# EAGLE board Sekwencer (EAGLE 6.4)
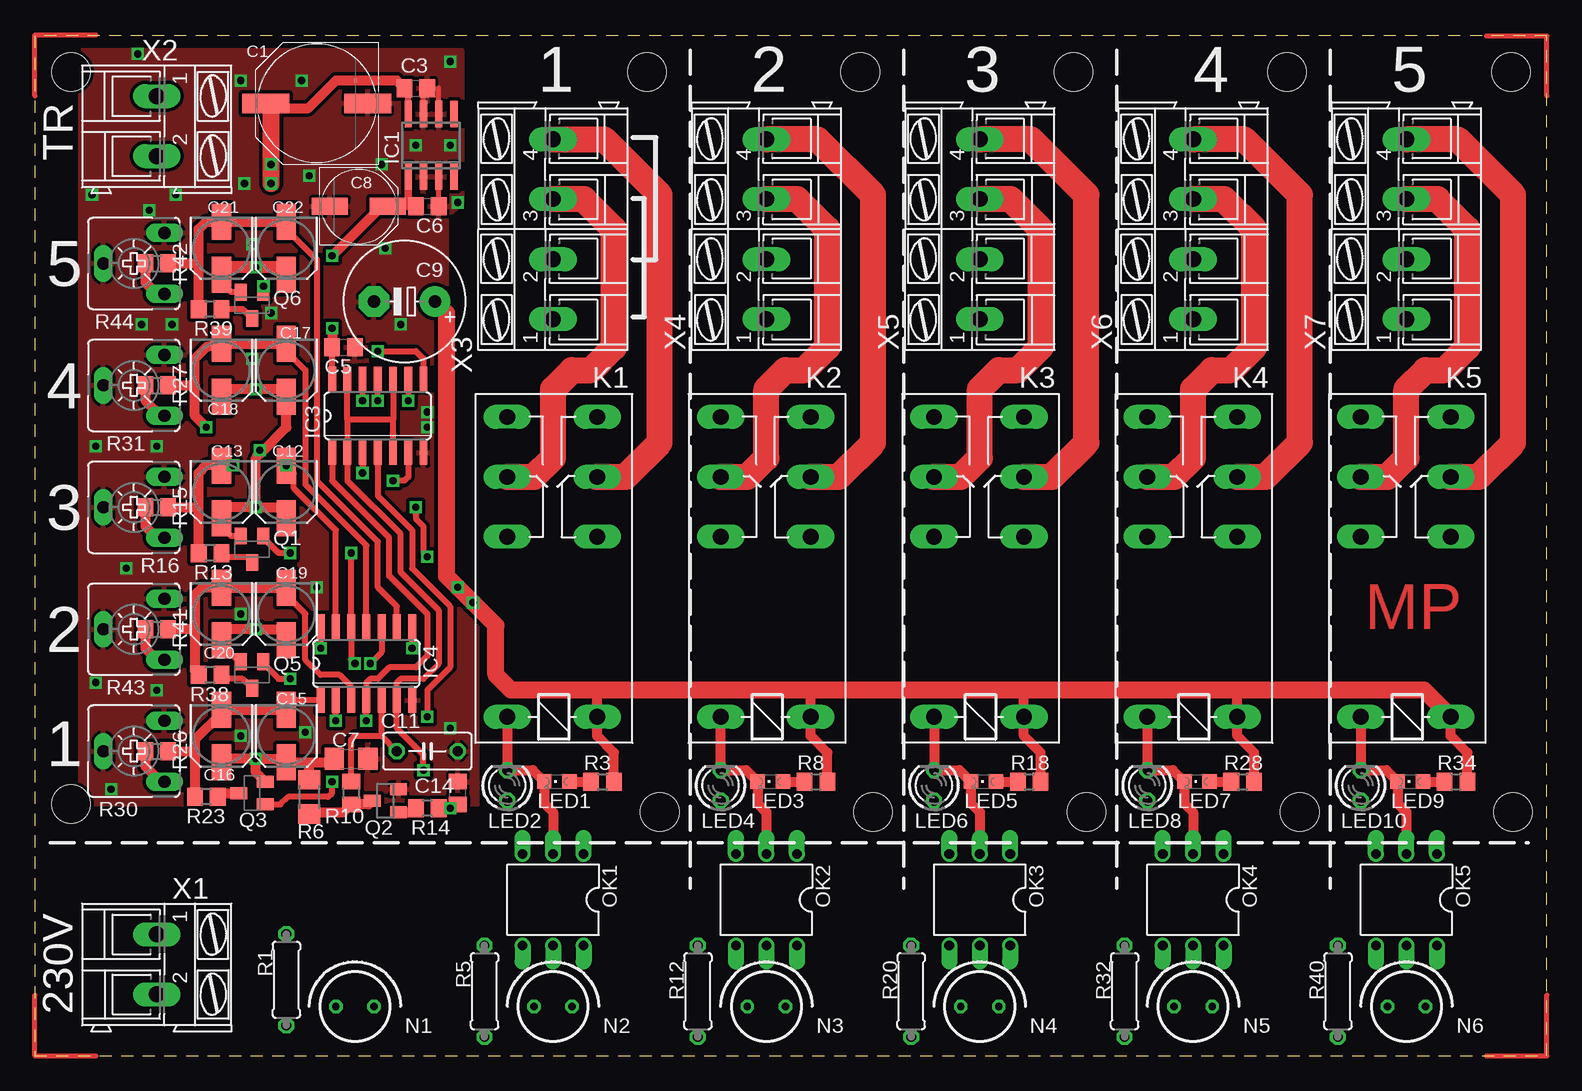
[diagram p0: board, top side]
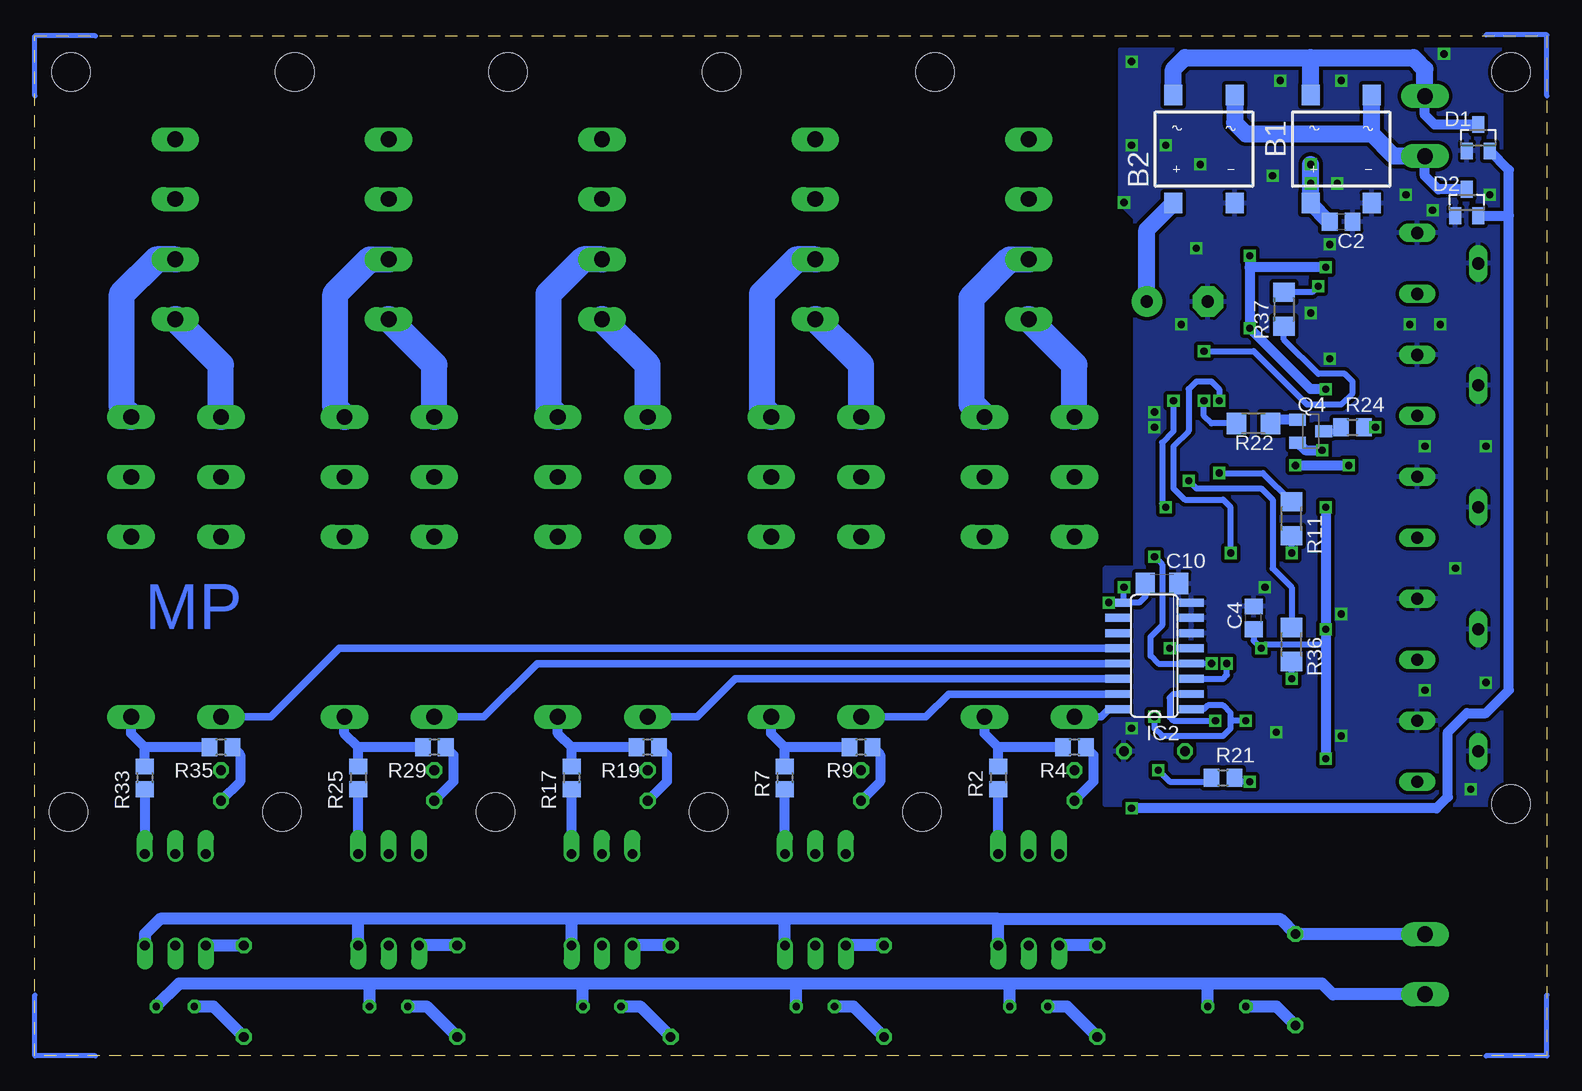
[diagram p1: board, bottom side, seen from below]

Size 126 x 85 mm. Coordinates in mm from the lower left corner, seen from the top.
Outline: 0,0 126,0 126,85 0,85 0,0
Copper layers (1*16): Top 0.035mm / dielectric 1.5mm / Bottom 0.035mm
Design rules "AVT-Elmax": minimum track width 8mil, minimum drill 18mil, track to track 8mil, track to pad 8mil, pad to pad 8mil, via to via 8mil, smd to smd 8mil, copper to edge 10mil, drill to drill 8mil, minimum pad ring 10mil, minimum via ring 8mil, stop-mask expansion 4mil, vias tented up to drill 0mil, thermal gap 10mil
Holes 3.2 mm at 52.07,20.32 69.85,20.32 87.63,20.32 105.41,20.32 123.19,20.32 51,82 68.78,82 86.56,82 104.34,82 123,82 3,82 3,21

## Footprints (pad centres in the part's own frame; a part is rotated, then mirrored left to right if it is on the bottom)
DFS = smd 1.5 x 1.7: + -2.55,-4.5; - 2.55,-4.5; AC1 -2.55,4.5; AC2 2.55,4.5
PANASONIC_G = smd 3.9 x 1.6: + 4.25,0; - -4.25,0
C0805 = smd 1.3 x 1.5: 1 -0.95,0; 2 0.95,0
C1206 = smd 1.6 x 1.8: 1 -1.4,0; 2 1.4,0
PANASONIC_D = smd 3 x 1.4: + 2.4,0; - -2.4,0
E5-10,5 = drill 1.016 pad 2.54: + -2.54,0 | drill 1.016 pad 2.54 octagon: - 2.54,0
C050-030X075 = drill 0.813 octagon: 1 -2.54,0; 2 2.54,0
SANYO-OSCON_SMD_B6 = smd 3 x 1.6: + 2.2,0; - -2.2,0
SOT23 = smd 1 x 1.4: 1 -0.95,-1.1; 2 0.95,-1.1; 3 0,1.1
SO-08 = smd 0.6 x 2.2: 1 -1.905,-2.6; 2 -0.635,-2.6; 3 0.635,-2.6; 4 1.905,-2.6; 5 1.905,2.6; 6 0.635,2.6; 7 -0.635,2.6; 8 -1.905,2.6
SO16 = smd 0.66 x 2.032: 1 -4.445,-3.073; 2 -3.175,-3.073; 3 -1.905,-3.073; 4 -0.635,-3.073; 5 0.635,-3.073; 6 1.905,-3.073; 7 3.175,-3.073; 8 4.445,-3.073; 9 4.445,3.073; 10 3.175,3.073; 11 1.905,3.073; 12 0.635,3.073; 13 -0.635,3.073; 14 -1.905,3.073; 15 -3.175,3.073; 16 -4.445,3.073
SO14 = smd 0.66 x 2.032: 1 -3.81,-3.073; 2 -2.54,-3.073; 3 -1.27,-3.073; 4 0,-3.073; 5 1.27,-3.073; 6 2.54,-3.073; 7 3.81,-3.073; 8 3.81,3.073; 9 2.54,3.073; 10 1.27,3.073; 11 0,3.073; 12 -1.27,3.073; 13 -2.54,3.073; 14 -3.81,3.073
G2R2 = drill 1.321 long: 1 -2.54,-3.683; 2 -2.54,3.81; O1 12.471,3.81; O2 12.471,-3.683; P1 17.45,3.81; P2 17.45,-3.683; S1 22.454,3.81; S2 22.454,-3.683
CHIPLED_0805 = smd 1.2 x 1.2: A 0,-1.05; C 0,1.05
LED3MM = drill 0.813 octagon: A -1.27,0; K 1.27,0
IN-3 = drill 0.6 octagon: A -1.587,0; K 1.587,0
DIL06 = drill 0.813 offset: 1 -2.54,-3.81; 2 0,-3.81; 3 2.54,-3.81; 4 2.54,3.81; 5 0,3.81; 6 -2.54,3.81
SOT23-BEC = smd 1 x 1.4: B -0.95,-1.1; C 0,1.1; E 0.95,-1.1
0207/7 = drill 0.813 octagon: 1 -3.81,0; 2 3.81,0
R0805 = smd 1.3 x 1.5: 1 -0.95,0; 2 0.95,0
R1206 = smd 1.6 x 1.803: 1 -1.422,0; 2 1.422,0
CA6V = drill 1.016 long: A -2.54,-2.54; E 2.54,-2.54; S 0,2.54
AK300/2 = drill 1.321 long: 1 -2.515,0; 2 2.489,0
AK300/4 = drill 1.321 long: 1 -7.493,0; 2 -2.515,0; 3 2.515,0; 4 7.493,0

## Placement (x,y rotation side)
B1  DF06S  [DFS]  17.14,75.56 0 bottom
B2  DF06S  [DFS]  28.57,75.56 0 bottom
C1  470u  [PANASONIC_G]  23.5,79.38 180 top
C2  100n  [C0805]  17.14,69.53 0 bottom
C3  100n  [C0805]  31.75,80.64 0 top
C4  100n  [C0805]  24.45,36.51 90 bottom
C5  100n  [C0805]  25.72,59.05 0 top
C6  100n  [C0805]  32.7,70.8 0 top
C7  100n  [C1206]  26.35,24.77 0 top
C8  100u  [PANASONIC_D]  26.99,70.8 0 top
C9  1000u  [E5-10,5]  30.8,62.87 180 top
C10  100n  [C1206]  32.07,39.37 0 bottom
C11  100n  [C050-030X075]  32.7,25.4 0 top
C12  22u  [SANYO-OSCON_SMD_B6]  20.95,46.99 270 top
C13  22u  [SANYO-OSCON_SMD_B6]  15.56,46.99 270 top
C14  100n  [C0805]  35.24,21.91 90 top
C15  22u  [SANYO-OSCON_SMD_B6]  20.95,26.67 270 top
C16  22u  [SANYO-OSCON_SMD_B6]  15.56,26.67 270 top
C17  22u  [SANYO-OSCON_SMD_B6]  20.95,57.15 270 top
C18  22u  [SANYO-OSCON_SMD_B6]  15.56,57.15 270 top
C19  22u  [SANYO-OSCON_SMD_B6]  20.95,36.83 270 top
C20  22u  [SANYO-OSCON_SMD_B6]  15.56,36.83 270 top
C21  22u  [SANYO-OSCON_SMD_B6]  15.56,67.31 270 top
C22  22u  [SANYO-OSCON_SMD_B6]  20.95,67.31 270 top
D1  BAV99  [SOT23]  5.71,76.52 0 bottom
D2  BAV99  [SOT23]  6.67,71.12 0 bottom
IC1  LM2931-5  [SO-08]  33.02,75.88 0 top
IC2  ULN2003  [SO16]  32.7,33.34 90 bottom
IC3  74HC08  [SO14]  28.57,53.34 0 top
IC4  74HC14  [SO14]  27.62,32.7 0 top
K1  RM83  [G2R2]  43.18,30.8 90 top
K2  RM83  [G2R2]  60.96,30.8 90 top
K3  RM83  [G2R2]  78.74,30.8 90 top
K4  RM83  [G2R2]  96.52,30.8 90 top
K5  RM83  [G2R2]  114.3,30.8 90 top
LED1  [CHIPLED_0805]  43.5,22.86 90 top
LED2  [LED3MM]  39.37,22.54 90 top
LED3  [CHIPLED_0805]  61.28,22.86 90 top
LED4  [LED3MM]  57.15,22.54 90 top
LED5  [CHIPLED_0805]  79.06,22.86 90 top
LED6  [LED3MM]  74.93,22.54 90 top
LED7  [CHIPLED_0805]  96.84,22.86 90 top
LED8  [LED3MM]  92.71,22.54 90 top
LED9  [CHIPLED_0805]  114.62,22.86 90 top
LED10  [LED3MM]  110.49,22.54 90 top
N1  IN-3  [IN-3]  26.67,4.13 0 top
N2  IN-3  [IN-3]  43.18,4.13 0 top
N3  IN-3  [IN-3]  60.96,4.13 0 top
N4  IN-3  [IN-3]  78.74,4.13 0 top
N5  IN-3  [IN-3]  96.52,4.13 0 top
N6  IN-3  [IN-3]  114.3,4.13 0 top
OK1  MOC3041M  [DIL06]  43.18,13.02 180 top
OK2  MOC3041M  [DIL06]  60.96,13.02 180 top
OK3  MOC3041M  [DIL06]  78.74,13.02 180 top
OK4  MOC3041M  [DIL06]  96.52,13.02 180 top
OK5  MOC3041M  [DIL06]  114.3,13.02 180 top
Q1  BC807-40  [SOT23-BEC]  18.1,42.23 180 top
Q2  BC846  [SOT23]  29.21,21.27 90 top
Q3  BC807-40  [SOT23-BEC]  18.1,21.91 90 top
Q4  BC807-40  [SOT23-BEC]  19.68,52.07 270 bottom
Q5  BC807-40  [SOT23-BEC]  18.1,31.75 180 top
Q6  BC807-40  [SOT23-BEC]  18.1,62.55 180 top
R1  220k  [0207/7]  20.95,6.35 270 top
R2  1k  [R0805]  45.72,23.18 270 bottom
R3  2k2  [R0805]  47.31,22.86 0 top
R4  *  [R0805]  39.37,25.72 180 bottom
R5  220k  [0207/7]  37.47,5.4 270 top
R6  51k  [R1206]  22.86,21.59 90 top
R7  1k  [R0805]  63.5,23.18 270 bottom
R8  2k2  [R0805]  65.09,22.86 0 top
R9  *  [R0805]  57.15,25.72 180 bottom
R10  100  [R0805]  26.35,21.91 270 top
R11  2k2  [R1206]  21.27,44.77 270 bottom
R12  220k  [0207/7]  55.24,5.4 270 top
R13  100  [R0805]  14.61,41.91 180 top
R14  10k  [R0805]  32.7,20.64 180 top
R15  10k  [R0805]  10.16,45.72 0 top
R16  1M  [CA6V]  8.26,45.72 90 top
R17  1k  [R0805]  81.28,23.18 270 bottom
R18  2k2  [R0805]  82.87,22.86 0 top
R19  *  [R0805]  74.93,25.72 180 bottom
R20  220k  [0207/7]  73.03,5.4 270 top
R21  2k2  [R0805]  26.99,23.18 0 bottom
R22  2k2  [R1206]  24.45,52.7 0 bottom
R23  100  [R0805]  14.29,21.59 180 top
R24  100  [R0805]  16.19,52.39 0 bottom
R25  1k  [R0805]  99.06,23.18 270 bottom
R26  10k  [R0805]  10.16,25.4 0 top
R27  10k  [R0805]  10.16,55.88 0 top
R28  2k2  [R0805]  100.65,22.86 0 top
R29  *  [R0805]  92.71,25.72 180 bottom
R30  1M  [CA6V]  8.26,25.4 90 top
R31  1M  [CA6V]  8.26,55.88 90 top
R32  220k  [0207/7]  90.81,5.4 270 top
R33  1k  [R0805]  116.84,23.18 270 bottom
R34  2k2  [R0805]  118.43,22.86 0 top
R35  *  [R0805]  110.49,25.72 180 bottom
R36  2k2  [R1206]  21.27,34.29 270 bottom
R37  2k2  [R1206]  21.91,62.23 90 bottom
R38  100  [R0805]  14.61,31.75 180 top
R39  100  [R0805]  14.61,62.23 180 top
R40  220k  [0207/7]  108.58,5.4 270 top
R41  10k  [R0805]  10.16,35.56 0 top
R42  10k  [R0805]  10.16,66.04 0 top
R43  1M  [CA6V]  8.26,35.56 90 top
R44  1M  [CA6V]  8.26,66.04 90 top
X1  230V  [AK300/2]  10.16,7.62 270 top
X2  TR  [AK300/2]  10.16,77.47 270 top
X3  [AK300/4]  43.18,68.9 90 top
X4  [AK300/4]  60.96,68.9 90 top
X5  [AK300/4]  78.74,68.9 90 top
X6  [AK300/4]  96.52,68.9 90 top
X7  [AK300/4]  114.3,68.9 90 top

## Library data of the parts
B1 B2 = rectifier
C1-C22 R1-R15 R17-R29 R32-R42 = rcl
D1 D2 = diode
IC1 = v-reg
IC2 = uln-udn
IC3 IC4 = 74xx-eu
K1-K5 = relay; MF: OMRON COMPONENTS USA; MPN: G2R-2-DC6; OC_FARNELL: unknown; OC_NEWARK: 89C5317
LED1-LED10 = led
N1-N6 = russian-nixies
OK1-OK5 = optocoupler; MF: FAIRCHILD SEMICONDUCTOR; MPN: MOC3041M; OC_FARNELL: 1086677; OC_NEWARK: 78K6090
Q1 Q3-Q6 = transistor-pnp
Q2 = transistor-npn
R16 R30 R31 R43 R44 = pot
X1-X7 = con-ptr500; OC_FARNELL: unknown; OC_NEWARK: unknown

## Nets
!RESET: IC3.2 IC3.5 IC3.10 IC3.13 IC4.6 R21.1
+5V: C4.1 C5.1 C6.1 C7.1 C8.+ C12.+ C13.+ C15.+ C16.+ C17.+ C18.+ C19.+ C20.+ C21.+ C22.+ IC1.1 IC3.14 IC4.14 Q1.E Q3.E Q4.E Q5.E Q6.E R6.2
GND: B1.- B2.- C1.- C2.2 C3.2 C4.2 C5.2 C6.2 C7.2 C8.- C9.- C10.2 C11.2 C14.2 D1.1 D2.1 IC1.2 IC1.3 IC1.6 IC1.7 IC2.6 IC2.7 IC2.8 IC3.7 IC4.7 Q2.2 R16.E R16.S R30.E R30.S R31.E R31.S R43.E R43.S R44.E R44.S
N$1: B1.AC1 B2.AC1 D1.3 X2.1
N$2: B1.AC2 B2.AC2 D2.3 X2.2
N$3: OK1.1 R2.2
N$4: K1.S1 X3.1
N$5: B1.+ C1.+ C2.1 C3.1 IC1.8
N$6: N1.A R1.2
N$7: LED1.A R3.1
N$8: LED2.A R4.1
N$9: Q2.1 R14.2
N$10: C14.1 D1.2 D2.2 R14.1
N$11: Q2.3 R6.1 R10.2
N$12: C15.- C16.- IC4.1 R23.2 R26.2
N$13: Q3.B R21.2
N$14: C19.- C20.- IC4.3 R38.2 R41.2
N$15: IC3.6 R36.1
N$16: Q5.B R36.2
N$17: R41.1 R43.A
N$18: IC3.3 R11.1
N$19: Q1.B R11.2
N$20: C12.- C13.- IC4.13 R13.2 R15.2
N$21: R15.1 R16.A
N$22: IC3.11 R22.1
N$23: Q4.B R22.2
N$24: C17.- C18.- IC4.11 R24.2 R27.2
N$25: R27.1 R31.A
N$26: Q6.B R37.2
N$27: C21.- C22.- IC4.9 R39.2 R42.2
N$28: R42.1 R44.A
N$29: IC3.8 R37.1
N$30: R26.1 R30.A
N$31: K1.P1 X3.3
N$32: K1.P2 X3.4
N$33: K1.S2 X3.2
N$34: OK1.4 R5.1
N$35: N2.A R5.2
N$36: K2.P2 X4.4
N$37: K2.S1 X4.1
N$38: K2.S2 X4.2
N$39: K2.P1 X4.3
N$40: OK2.4 R12.1
N$41: N3.A R12.2
N$42: LED4.A R9.1
N$43: LED3.A R8.1
N$45: OK2.1 R7.2
N$46: OK3.1 R17.2
N$47: K3.S1 X5.1
N$48: LED6.A R19.1
N$49: LED5.A R18.1
N$50: K4.P2 X6.4
N$52: OK3.4 R20.1
N$53: N4.A R20.2
N$54: K3.P2 X5.4
N$55: K3.S2 X5.2
N$56: K3.P1 X5.3
N$57: K4.S1 X6.1
N$58: K4.S2 X6.2
N$59: K4.P1 X6.3
N$60: OK4.4 R32.1
N$61: N5.A R32.2
N$62: LED8.A R29.1
N$63: LED7.A R28.1
N$65: OK4.1 R25.2
N$66: OK5.1 R33.2
N$67: LED10.A R35.1
N$68: LED9.A R34.1
N$70: OK5.4 R40.1
N$71: N6.A R40.2
N$72: K5.P2 X7.4
N$73: K5.S2 X7.2
N$74: K5.P1 X7.3
N$75: K5.S1 X7.1
N$76: N1.K N2.K N3.K N4.K N5.K N6.K X1.2
N$77: OK1.6 OK2.6 OK3.6 OK4.6 OK5.6 R1.1 X1.1
N$82: Q6.C R39.1
N$83: Q4.C R24.1
N$84: Q1.C R13.1
N$85: Q5.C R38.1
N$86: Q3.C R23.1
N$87: C11.1 IC4.5 R10.1
OC1: IC2.16 K1.2 LED1.C LED2.K OK1.2
OC2: IC2.15 K2.2 LED3.C LED4.K OK2.2
OC3: IC2.14 K3.2 LED5.C LED6.K OK3.2
OC4: IC2.13 K4.2 LED7.C LED8.K OK4.2
OC5: IC2.12 K5.2 LED9.C LED10.K OK5.2
REL1: IC2.1 IC3.4 IC4.2
REL2: IC2.2 IC3.1 IC4.4
REL3: IC2.3 IC3.12 IC4.12
REL4: IC2.4 IC3.9 IC4.10
REL5: IC2.5 IC4.8
VCC: B2.+ C9.+ C10.1 IC2.9 K1.1 K2.1 K3.1 K4.1 K5.1 R2.1 R3.2 R4.2 R7.1 R8.2 R9.2 R17.1 R18.2 R19.2 R25.1 R28.2 R29.2 R33.1 R34.2 R35.2

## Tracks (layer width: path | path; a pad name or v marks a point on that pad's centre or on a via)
!RESET  (via drill 0.6)
  Top 0.508: 26.04,53.02 IC3.13 | IC3.10 29.84,53.02 | 29.84,53.02 26.04,53.02 | IC3.5 29.84,53.02 | 26.04,53.02 IC3.2 26.04,47.94 30.48,43.5 30.48,40.32 33.66,37.15 33.66,32.7 32.38,31.43 30.48,31.43 30.16,31.11 IC4.6 30.16,27.3 32.38,25.08 v32.38,23.81
  Bottom 0.508: v32.38,23.81 31.43,22.86 28.25,22.86 R21.1
+5V  (via drill 0.6, 0.6 pad 0.25)
  Top 0.508: IC4.14 v23.81,33.97 | IC3.14 C5.1 | Q1.E 16.36,43.33 15.56,44.13 C13.+ | Q5.E 17,32.85 15.56,34.29 C20.+ | Q6.E 16.36,63.65 15.56,64.45 C21.+
  Top 0.61: C8.+ 31.11,70.8 | 31.11,70.8 C6.1 | IC1.1 31.11,70.8
  Top 0.813: v24.77,60.64 C5.1 | 18.41,45.71 v18.41,45.72 18.41,49.85 18.89,50.32 | v18.41,55.55 v18.41,55.56 | v24.77,66.67 28.89,70.8 C8.+ | v18.41,55.56 15.85,55.56 C18.+ | v18.41,55.56 20.66,55.56 C17.+ 20.95,52.39 18.89,50.32 | 18.41,45.71 15.56,45.71 C13.+ | 18.41,45.71 20.95,45.71 C12.+ | v18.73,50.48 18.89,50.32 | C20.+ 15.56,35.55 v18.41,35.55 20.95,35.55 C19.+ | v18.41,24.77 15.85,24.77 C16.+ | v18.41,24.77 20.02,24.77 C15.+ 22.86,24.47 | 22.86,24.47 24.66,24.47 C7.1 | R6.2 22.86,24.47 | Q3.E 18.41,23.64 v18.41,24.77
  Top 1.016: C22.+ 20.93,65.72 v18.41,65.72 15.58,65.72 C21.+
  Bottom 0.508: 18.41,33.97 18.41,34.29 23.5,34.29 v23.81,33.97 24.45,34.61 C4.1 | Q4.E
  Bottom 0.813: v24.77,66.67 24.77,65.72 | 24.77,65.72 v24.77,60.64 19.68,55.56 v18.41,55.56 | v18.41,45.72 v18.41,35.55 18.41,33.97 v18.41,24.77 | v18.41,65.72 24.77,65.72 | Q4.E 20.15,50.48 v18.73,50.48
GND  (via drill 0.6)
  Top 0.406: 33.66,78.42 33.66,80.64 | 32.38,78.74 32.38,80.64 | 33.66,71.12 33.66,73.03
  other vias: 32.7,53.66 32.7,52.39 5.08,31.11 10.16,30.48 7.62,40.64 5.08,50.8 10.16,50.8 8.89,60.96 11.43,60.96 9.53,70.48 29.21,67.31 30.48,60.96 28.89,74.3 34.61,82.87 22.23,81.28 22.54,26.99 11.75,71.75 34.61,75.88 31.75,75.88 34.61,27.3 17.46,72.71 17.14,81.28 22.86,73.34 18.1,67.63 8.57,83.5 35.24,71.12 4.76,71.75 6.35,22.23 19.68,61.91 18.1,58.1 23.5,39.05 17.14,36.83 17.14,26.67
  pour Top (isolate 0.305): 3.81,83.82 35.56,83.82 35.56,71.12 34.29,69.85 34.29,40.64 36.83,40.64 36.83,20.95 3.81,20.95
  pour Bottom (isolate 0.305): 3.81,83.82 35.56,83.82 35.56,71.12 34.29,69.85 34.29,40.64 36.83,40.64 36.83,20.95 3.81,20.95
N$1
  Bottom 0.813: 9.99,82.06 10.16,82.23 | D1.3 9.36,77.62 10.16,78.42 X2.1
  Bottom 1.422: X2.1 10.16,82.23 11.11,83.19 19.68,83.19 | B2.AC1 31.12,82.22 30.16,83.19 19.68,83.19 | B1.AC1 19.7,82.54 19.68,83.19
N$2
  Bottom 0.813: D2.3 9.04,72.22 10.16,73.34 X2.2
  Bottom 1.422: X2.2 12.75,74.98 14.61,76.83 | 14.61,76.83 14.61,80.06 B1.AC2 | B2.AC2 26.02,77.78 25.08,76.83 14.61,76.83
N$3
  Bottom 0.813: OK1.1 R2.2
N$4
  Bottom 2.184: K1.S1 39.37,57.59 X3.1
N$5  (via drill 0.6)
  Top 0.508: IC1.8 31.11,80.33 C3.1
  Top 0.813: C3.1 30.16,81.28 25.08,81.28 22.74,78.94 19.68,78.94
  Top 1.422: v19.68,72.71 v19.68,74.3 19.68,78.94 C1.+
  Bottom 1.27: C2.1 18.16,69.53 B1.+
  Bottom 1.422: B1.+ 19.7,72.08 v19.68,72.71 v19.68,74.3
N$6
  Bottom 1.016: N1.A 22.54,4.13 R1.2
N$7
  Top 0.813: LED1.A R3.1
N$8
  Bottom 0.813: R4.1 37.78,25.08 37.78,22.86 LED2.A
N$9
  Top 0.813: Q2.1 31.44,20.32 R14.2
N$10  (via drill 0.6)
  Top 0.508: R14.1 33.65,20.32
  Top 0.813: 33.65,20.32 33.66,20.32 | R14.1 v34.61,20.64 34.93,20.96 C14.1
  Bottom 0.813: v34.61,20.64 9.21,20.64 8.26,21.59 8.26,26.99 6.67,28.57 5.08,28.57 3.17,30.48 3.17,70.02 | 3.17,70.02 3.17,73.83 D1.2 | D2.2 3.17,70.02
N$11
  Top 0.813: R6.1 23.01,20.32 25.71,20.32 R10.2 27.8,20.96 Q2.3
N$12
  Top 0.508: IC4.1 21.06,29.63 20.32,28.89 C15.-
  Top 0.813: C15.- C16.- 15.56,28.57 13.34,26.35 13.34,25.4 | 13.34,25.4 13.34,22.86 R23.2 | R26.2 13.34,25.4
N$13  (via drill 0.6)
  Top 0.508: v24.77,22.86 24.77,21.91 24.45,21.59 21.1,21.59 20.47,20.96 Q3.B
  Bottom 0.508: v24.77,22.86 25.72,22.86 R21.2
N$14
  Top 0.508: IC4.3 26.35,30.8 25.4,31.75 23.81,31.75 22.54,33.02 22.54,36.83 20.95,38.42 C19.-
  Top 0.813: C19.- C20.- 13.95,39.03 13.34,38.42 13.34,35.56 | 13.34,35.56 R41.2 | 13.34,35.56 13.34,32.07 R38.2
N$15  (via drill 0.6)
  Top 0.508: IC3.6 31.11,48.26 30.8,47.94 v29.84,47.94
  Bottom 0.508: R36.1 21.27,39.05 22.86,40.64 22.86,46.35 23.81,47.31 29.21,47.31 v29.84,47.94
N$16  (via drill 0.6)
  Top 0.508: Q5.B 19.05,32.7 20.32,31.43 v21.27,31.43
  Bottom 0.508: v21.27,31.43 R36.2
N$17
  Top 0.813: R41.1 9.21,33.97 10.16,33.02 R43.A
N$18  (via drill 0.6)
  Top 0.508: IC3.3 v27.3,48.58
  Bottom 0.508: v27.3,48.58 23.66,48.58 R11.1
N$19  (via drill 0.6)
  Top 0.508: Q1.B 19.05,43.18 20.32,41.91 v21.27,41.91
  Bottom 0.508: v21.27,41.91 R11.2
N$20  (via drill 0.6)
  Top 0.508: IC4.13 25.08,43.81 21.59,47.31 21.59,48.55 C12.-
  Top 0.813: C13.- 14.3,49.23 13.65,48.58 13.65,45.72 | 15.57,48.9 C13.- | v20.95,49.21 20.62,49.21 C12.- | v16.51,49.21 15.86,49.21 C13.- | R15.2 13.65,45.72 | R13.2 13.65,45.72
  Bottom 0.813: v20.95,49.21 v16.51,49.21
N$21
  Top 0.813: R15.1 9.21,44.13 10.16,43.18 R16.A
N$22  (via drill 0.6)
  Top 0.508: v28.57,54.61 IC3.11
  Bottom 0.508: v28.57,54.61 28.57,53.34 27.94,52.7 R22.1
N$23
  Bottom 0.813: Q4.B 22.71,53.02 R22.2
N$24  (via drill 0.6 pad 0.25)
  Top 0.508: IC4.11 27.62,42.55 22.54,47.62 22.54,57.15 20.95,58.74 C17.-
  Top 0.813: C17.- C18.- 14.3,59.07 13.34,58.1 13.34,55.88 | v14.29,52.39 13.34,53.34 13.34,55.88 | R27.2 13.34,55.88
  Bottom 0.813: R24.2 v14.29,52.39
N$25
  Top 0.813: R27.1 9.21,54.61 10.48,53.34 R31.A
N$26  (via drill 0.6 pad 0.25)
  Top 0.508: Q6.B v19.05,64.14
  Bottom 0.508: v19.05,64.14 19.53,63.65 R37.2
N$27
  Top 0.508: IC4.9 30.16,37.47 28.57,39.05 28.57,42.86 23.5,47.94 23.5,66.36 20.95,68.9 C22.-
  Top 0.813: C22.- C21.- 14.27,69.51 13.65,68.9 13.65,66.04 | R39.2 13.65,66.04 | R42.2 13.65,66.04
N$28
  Top 0.813: R42.1 9.21,64.45 10.16,63.5 R44.A
N$29  (via drill 0.6)
  Top 0.508: v28.57,58.74 31.75,58.74 32.38,58.1 IC3.8
  Bottom 0.508: v28.57,58.74 24.45,58.74 20,54.29 17.14,54.29 16.19,55.24 16.19,56.2 16.83,56.83 19.05,56.83 21.91,59.69 R37.1
N$30
  Top 0.813: R26.1 9.21,24.13 10.48,22.86 R30.A
N$31
  Top 2.184: K1.P1 41.58,48.25 43.18,49.85 43.18,55.56 44.77,57.15 46.35,57.15 48.26,59.05 48.26,68.9 45.74,71.41 X3.3
N$32
  Top 2.184: K1.P2 49.2,48.25 52.07,51.12 52.07,71.75 47.43,76.39 X3.4
N$33
  Bottom 2.184: K1.S2 47.94,54.33 47.94,63.18 44.74,66.38 X3.2
N$34
  Bottom 1.016: R5.1 OK1.4
N$35
  Bottom 1.016: N2.A 40.01,4.13 R5.2
N$36
  Top 2.184: K2.P2 66.98,48.25 69.85,51.12 69.85,71.75 65.22,76.39 X4.4
N$37
  Bottom 2.184: K2.S1 57.15,57.59 X4.1
N$38
  Bottom 2.184: K2.S2 65.41,54.01 65.41,63.5 62.52,66.38 X4.2
N$39
  Top 2.184: K2.P1 59.36,48.25 60.96,49.85 60.96,55.56 62.55,57.15 64.14,57.15 66.04,59.05 66.04,68.9 63.52,71.41 X4.3
N$40
  Bottom 1.016: R12.1 OK2.4
N$41
  Bottom 1.016: N3.A 57.78,4.13 R12.2
N$42
  Bottom 0.813: R9.1 55.56,25.08 55.56,22.86 LED4.A
N$43
  Top 0.813: LED3.A R8.1
N$44
  Bottom 0.406: 0,80.01 0,85.09 5.08,85.09
N$45
  Bottom 0.813: OK2.1 R7.2
N$46
  Bottom 0.813: OK3.1 R17.2
N$47
  Bottom 2.184: K3.S1 74.93,57.59 X5.1
N$48
  Bottom 0.813: R19.1 73.34,25.08 73.34,22.86 LED6.A
N$49
  Top 0.813: LED5.A R18.1
N$50
  Top 2.184: K4.P2 102.54,48.25 105.41,51.12 105.41,71.75 100.78,76.39 X6.4
N$51
  Bottom 0.406: 120.97,0 126,0 126,5.08
N$52
  Bottom 1.016: R20.1 OK3.4
N$53
  Bottom 1.016: N4.A 75.56,4.13 R20.2
N$54
  Top 2.184: K3.P2 84.76,48.25 87.63,51.12 87.63,71.75 83,76.39 X5.4
N$55
  Bottom 2.184: K3.S2 83.19,54.01 83.19,63.5 80.3,66.38 X5.2
N$56
  Top 2.184: K3.P1 77.14,48.25 78.74,49.85 78.74,55.56 80.33,57.15 81.92,57.15 83.82,59.05 83.82,68.9 81.31,71.41 X5.3
N$57
  Bottom 2.184: K4.S1 92.71,57.59 X6.1
N$58
  Bottom 2.184: K4.S2 100.97,54.01 100.97,63.5 98.08,66.38 X6.2
N$59
  Top 2.184: K4.P1 94.92,48.25 96.52,49.85 96.52,55.56 98.11,57.15 99.69,57.15 101.6,59.05 101.6,68.9 99.08,71.41 X6.3
N$60
  Bottom 1.016: R32.1 OK4.4
N$61
  Bottom 1.016: N5.A 93.34,4.13 R32.2
N$62
  Bottom 0.813: R29.1 91.12,25.08 91.12,22.86 LED8.A
N$63
  Top 0.813: LED7.A R28.1
N$64
  Top 0.406: 126,80.01 126,85 120.97,85
N$65
  Bottom 0.813: OK4.1 R25.2
N$66
  Bottom 0.813: R33.2 OK5.1
N$67
  Bottom 0.813: R35.1 108.9,25.08 108.9,22.86 LED10.A
N$68
  Top 0.813: LED9.A R34.1
N$69
  Top 0.406: 0,80.01 0,85.09 5.08,85.09
N$70
  Bottom 1.016: OK5.4 R40.1
N$71
  Bottom 1.016: N6.A 111.12,4.13 R40.2
N$72
  Top 2.184: K5.P2 120.32,48.25 123.19,51.12 123.19,71.75 118.56,76.39 X7.4
N$73
  Bottom 2.184: K5.S2 118.75,54.01 118.75,63.5 115.86,66.38 X7.2
N$74
  Top 2.184: K5.P1 112.7,48.25 114.3,49.85 114.3,55.56 115.89,57.15 117.47,57.15 119.38,59.05 119.38,68.9 116.86,71.41 X7.3
N$75
  Bottom 2.184: K5.S1 110.49,57.59 X7.1
N$76
  Bottom 1.016: X1.2 17.83,5.13 18.73,6.03 28.26,6.03 | 28.26,6.03 44.77,6.03 | 44.77,6.03 62.55,6.03 | 62.55,6.03 80.33,6.03 | 80.33,6.03 98.11,6.03 | 98.11,6.03 113.98,6.03 N6.K | N5.K 98.11,6.03 | N4.K 80.33,6.03 | N3.K 62.55,6.03 | N2.K 44.77,6.03 | N1.K 28.26,6.03
N$77
  Bottom 1.016: 45.72,11.43 63.5,11.43 | 63.5,11.43 81.28,11.43 | 81.28,11.43 99.06,11.43 | 99.06,11.43 115.57,11.43 116.84,10.16 OK5.6 | OK4.6 99.06,11.43 | OK3.6 81.28,11.43 | OK2.6 63.5,11.43 | OK1.6 45.72,11.43 | X1.1 20.95,10.13 R1.1 22.23,11.43 45.72,11.43
N$78
  Top 0.406: 0,5.08 0,0 5.08,0
N$79
  Top 0.406: 120.97,0 126,0 126,5.08
N$80
  Bottom 0.406: 0,5.08 0,0 5.08,0
N$81
  Bottom 0.406: 126,80.01 126,85 120.97,85
N$82
  Top 0.508: Q6.C 17.32,62.23 R39.1
N$83
  Bottom 0.508: Q4.C 17.46,52.07 R24.1
N$84
  Top 0.508: R13.1 15.87,41.59 17.63,41.59 Q1.C
N$85
  Top 0.508: Q5.C 17.32,31.43 15.87,31.43 R38.1
N$86
  Top 0.813: R23.1 15.55,21.91 Q3.C
N$87
  Top 0.508: 28.89,26.67 IC4.5 | 28.89,26.67 26.67,26.67 26.35,26.35 R10.1 | 28.89,26.67 C11.1
OC1
  Top 0.813: K1.2 LED2.K 41.49,23.81 LED1.C 42.45,21.05 43.18,20.32 OK1.2
  Bottom 0.61: K1.2 37.15,28.26 36.51,28.89 IC2.16
OC2
  Top 0.813: OK2.2 60.96,20.32 60.23,21.05 LED3.C 59.27,23.81 LED4.K K2.2
  Bottom 0.61: IC2.15 49.85,30.16 51.75,28.26 K2.2
OC3
  Top 0.813: OK3.2 78.74,20.32 78.01,21.05 LED5.C 77.06,23.81 LED6.K K3.2
  Bottom 0.61: IC2.14 67.63,31.43 70.8,28.26 K3.2
OC4
  Top 0.813: OK4.2 96.52,20.32 95.79,21.05 LED7.C 94.83,23.81 LED8.K K4.2
  Bottom 0.61: IC2.13 84.14,32.7 88.58,28.26 K4.2
OC5
  Top 0.813: OK5.2 114.3,20.32 113.57,21.05 LED9.C 112.61,23.81 LED10.K K5.2
  Bottom 0.61: IC2.12 100.65,33.97 106.36,28.26 K5.2
REL1  (via drill 0.6)
  Top 0.508: v25.08,27.94 IC4.2 | IC3.4 28.57,46.67 31.43,43.81 31.43,40.64 34.61,37.47 34.61,32.38 32.7,30.48 v32.7,28.26
  Bottom 0.508: IC2.1 28.57,28.89 28.26,29.21 26.99,29.21 26.35,28.57 26.35,27.94 | v32.7,28.26 32.7,27.3 32.07,26.67 26.99,26.67 26.35,27.3 26.35,27.94 | v25.08,27.94 26.35,27.94
REL2  (via drill 0.6)
  Top 0.508: v27.62,27.94 IC4.4 27.62,31.11 27.94,31.43 28.57,31.43 29.53,32.38 31.75,32.38 32.7,33.34 32.7,36.83 29.53,40.01 29.53,43.18 24.77,47.94 IC3.1
  Bottom 0.508: IC2.2 31.11,30.16 31.43,29.84 31.43,28.26 31.11,27.94 v27.62,27.94
REL3  (via drill 0.6)
  Top 0.508: v26.35,41.91 IC4.12 26.35,33.02 v26.67,32.7 | v27.3,54.61 IC3.12
  Bottom 0.508: IC2.3 26.99,31.43 26.67,31.75 v26.67,32.7 | v26.35,41.91 26.35,45.72 26.99,46.35 30.16,46.35 31.11,47.31 31.11,50.8 29.84,52.07 29.84,55.56 29.21,56.2 27.94,56.2 27.3,55.56 v27.3,54.61
REL4  (via drill 0.6)
  Top 0.508: IC4.10 28.89,33.66 v27.94,32.7 | IC3.9 v31.11,54.61 | v31.75,45.72 31.75,44.77 32.38,44.13 32.38,41.91 v32.7,41.59
  Bottom 0.508: v27.94,32.7 IC2.4 32.38,32.7 33.02,33.34 33.02,34.92 32.07,35.88 32.07,40.96 v32.7,41.59 | v31.11,54.61 31.11,52.07 32.07,51.12 32.07,46.04 v31.75,45.72
REL5  (via drill 0.6)
  Top 0.508: v31.43,33.97 IC4.8
  Bottom 0.508: IC2.5 v31.43,33.97
VCC  (via drill 0.6)
  Top 0.813: R3.2 48.26,25.28 46.86,26.67 K1.1 46.86,30.35 46.99,30.48 | R8.2 66.04,25.28 64.64,26.67 K2.1 64.64,30.35 64.77,30.48 | R18.2 83.82,25.28 82.42,26.67 K3.1 82.42,30.35 82.55,30.48 | R28.2 101.6,25.28 100.2,26.67 K4.1 100.2,30.35 100.33,30.48 | R34.2 119.38,25.28 117.98,26.67 K5.1
  Top 1.422: C9.+ 34.29,61.91 34.29,40.01 v35.24,39.05 v36.51,37.78 38.42,35.88 38.42,31.75 39.69,30.48 46.99,30.48 64.77,30.48 82.55,30.48 100.33,30.48 115.76,30.48 K5.1
  Bottom 0.508: v36.51,37.78 IC2.9 35.24,37.78 | 35.24,37.78 v35.24,39.05 | C10.1 33.47,38.29 33.97,37.78 35.24,37.78
  Bottom 0.61: 35.88,37.78 IC2.9
  Bottom 0.813: R4.2 45.72,25.72 | 45.72,25.72 46.86,26.86 K1.1 | R9.2 63.5,25.72 | 63.5,25.72 64.64,26.86 K2.1 | R19.2 81.28,25.72 | 81.28,25.72 82.42,26.86 K3.1 | R29.2 99.06,25.72 | 99.06,25.72 100.2,26.86 K4.1 | R35.2 116.84,25.72 | 116.84,25.72 117.98,26.86 K5.1 | R2.1 45.72,25.72 | R7.1 63.5,25.72 | R17.1 81.28,25.72 | R25.1 99.06,25.72 | R33.1 116.84,25.72
  Bottom 1.422: C9.+ 33.34,68.85 B2.+

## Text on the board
Top: MP
Bottom: MP
tPlace: 1 | 2 | 3 | 4 | 5 | TR | 5 | 4 | 3 | 2 | 1 | 230V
